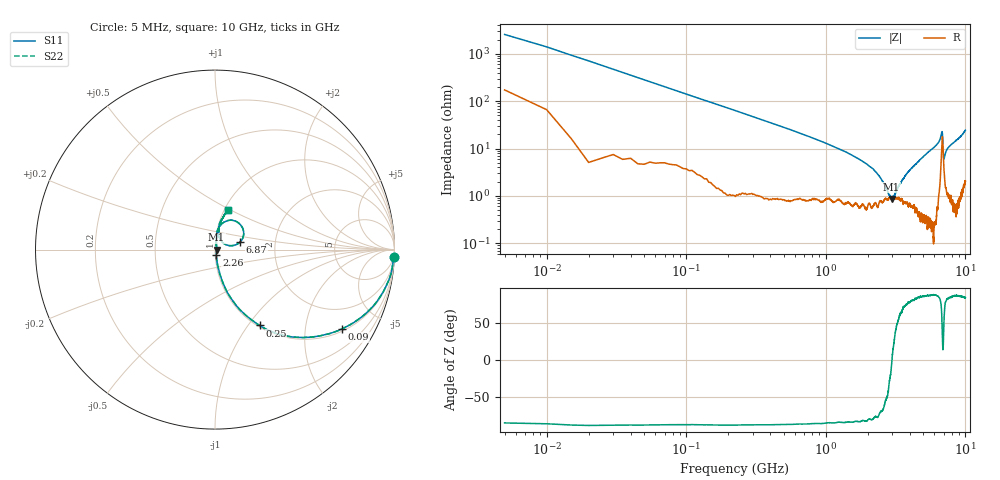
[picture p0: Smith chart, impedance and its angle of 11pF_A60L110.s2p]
! Amotech Co.,Ltd.
! http://www.amotech.co.kr/
! Part Number: A60L110
! These Parameters are Measured in Series Mode Connection
! Operation Temp=25[degC], DC Bias Voltage=0[V]
! Freq. Start=5[MHz] Stop=10[GHz], 2000[Steps]
! Date: Monday, July 14, 2020, 10:04:15
# GHZ S RI R 50.000000
!Freq.(Hz) S11(Real) S11(Imag) S21(Real) S21(Imag) S12(Real) S12(Imag) S22(Real) S22(Imag)
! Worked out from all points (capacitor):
!   2000 points, 5 MHz to 10 GHz, reference 50 ohm
!   read as one part in series: C = 11.2 pF near 55 MHz
!   lowest |Z| = 867 mohm at 2.96 GHz (marker M1)
!   series resonance near 2.979 GHz, so ESL is about 250 pH
!   S11 on the Smith chart (normalised r, x): 5 MHz: 4, -51; 90 MHz: 1.08, -3.15; 250 MHz: 1.02, -1.14; 2.26 GHz: 1.01, -0.06; 6.87 GHz: 1.32, +0.12; 10 GHz: 1.04, +0.49
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0.005  0.9959 -0.0385  0.0041 0.0385  0.0041 0.0385  0.9959 -0.0385
0.06  0.8433 -0.3533  0.1567 0.3533  0.1567 0.3533  0.8433 -0.3533
0.09  0.7073 -0.442  0.2927 0.442  0.2927 0.442  0.7073 -0.442
0.15  0.4743 -0.4894  0.5257 0.4894  0.5257 0.4894  0.4743 -0.4894
0.25  0.2493 -0.4227  0.7507 0.4227  0.7507 0.4227  0.2493 -0.4227
0.385  0.1249 -0.319  0.8751 0.319  0.8751 0.319  0.1249 -0.319
0.595  0.0588 -0.2181  0.9412 0.2181  0.9412 0.2181  0.0588 -0.2181
1.675  0.0106 -0.0617  0.9894 0.0617  0.9894 0.0617  0.0106 -0.0617
2.26  0.00818 -0.0315  0.9918 0.0315  0.9918 0.0315  0.00818 -0.0315
2.96  0.00853 -0.00102  0.9915 0.00102  0.9915 0.00102  0.00853 -0.00102
3.34  0.00926 0.0138  0.9907 -0.0138  0.9907 -0.0138  0.00926 0.0138
3.855  0.0076 0.0299  0.9924 -0.0299  0.9924 -0.0299  0.0076 0.0299
5.005  0.00789 0.0669  0.9921 -0.0669  0.9921 -0.0669  0.00789 0.0669
6.375  0.0228 0.1268  0.9772 -0.1268  0.9772 -0.1268  0.0228 0.1268
6.67  0.0631 0.159  0.9369 -0.159  0.9369 -0.159  0.0631 0.159
6.795  0.1424 0.1375  0.8576 -0.1375  0.8576 -0.1375  0.1424 0.1375
6.87  0.1409 0.0434  0.8591 -0.0434  0.8591 -0.0434  0.1409 0.0434
6.96  0.0603 0.0277  0.9397 -0.0277  0.9397 -0.0277  0.0603 0.0277
7.02  0.0381 0.0438  0.9619 -0.0438  0.9619 -0.0438  0.0381 0.0438
7.405  0.0195 0.0939  0.9805 -0.0939  0.9805 -0.0939  0.0195 0.0939
8.335  0.0234 0.1346  0.9766 -0.1346  0.9766 -0.1346  0.0234 0.1346
10  0.0735 0.2223  0.9265 -0.2223  0.9265 -0.2223  0.0735 0.2223
